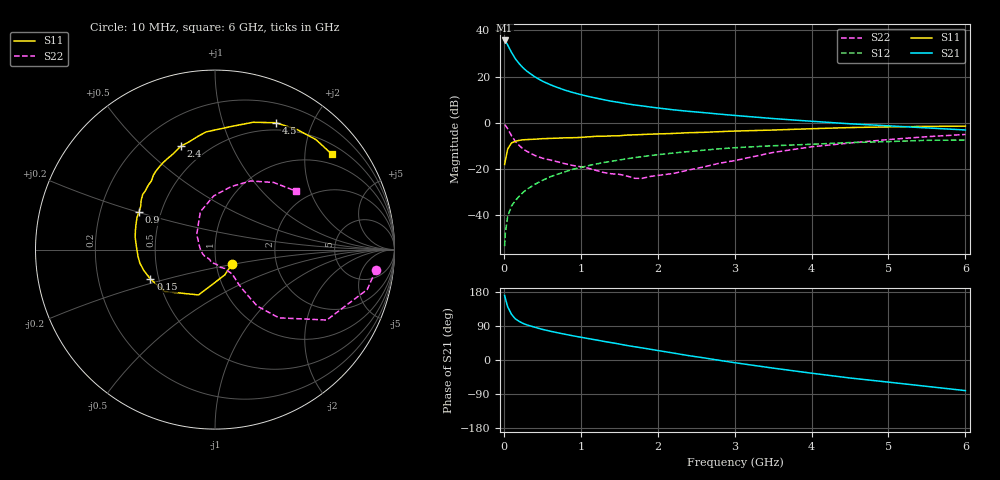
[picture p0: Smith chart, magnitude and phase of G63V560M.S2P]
! SIEMENS Small Signal Semiconductors
! BFG193
! Si NPN RF Bipolar Junction Transistor in SOT223
! VCE = 3.5 V  IC = 60 mA
! Common Emitter S-Parameters:  August  1996
# GHz  S  MA  R  50
!  f  S11  S21  S12  S22
! GHz  MAG  ANG  MAG  ANG  MAG  ANG  MAG  ANG
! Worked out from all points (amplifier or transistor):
!   36 points, 10 MHz to 6 GHz, reference 50 ohm
!   highest |S21| = 35.7 dB at 10 MHz (marker M1)
!   |S21| within 3 dB of that: start of sweep to 65.8 MHz
!   unconditionally stable (mu >= 1): 374.2 MHz to 2.36 GHz
!   at 250 MHz: K = 0.94, MSG = 27.0 dB, |S12| = -30.2 dB
!   at 1.4 GHz: K = 1.05, MAG = 11.7 dB, |S12| = -16.7 dB
!   at 6 GHz: K = 0.90, MSG = 2.2 dB, |S12| = -7.5 dB
!   S11 on the Smith chart (normalised r, x): 10 MHz: 1.20, -0.19; 150 MHz: 0.45, -0.17; 900 MHz: 0.37, +0.20; 2.4 GHz: 0.36, +0.66; 4.5 GHz: 0.41, +1.51; 6 GHz: 0.72, +2.62
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0.01  0.1243 -38.9  60.7 170.5  0.0021 85.1  0.904 -7.2
0.02  0.1516 -69.2  58.49 162.1  0.0041 80.7  0.8767 -14.7
0.05  0.2685 -109.9  48.3 140.4  0.0093 73.3  0.7363 -32.2
0.1  0.3646 -140.2  33.37 120.5  0.0156 69.3  0.5208 -46.9
0.15  0.3951 -155.5  24.27 108.4  0.0205 67.5  0.3926 -53.2
0.2  0.4136 -163.7  19.03 101.8  0.0254 70.7  0.3212 -54.3
0.25  0.4253 -169.8  15.48 96.5  0.0309 69.8  0.2679 -55.2
0.3  0.4305 -174.8  13.08 92.6  0.0359 70.5  0.2393 -55.7
0.4  0.4379 178.0  9.943 86.6  0.0458 70.7  0.1954 -55.2
0.5  0.4499 171.3  7.975 80.9  0.0559 69.6  0.1703 -54.9
0.6  0.4562 166.5  6.707 76.2  0.0668 68.4  0.1555 -56.1
0.7  0.4623 162.1  5.77 71.8  0.0765 66.8  0.1419 -58.6
0.9  0.4728 153.7  4.503 63.8  0.0978 63.1  0.1179 -62.6
1.1  0.4935 146.6  3.703 56.5  0.1173 59.6  0.1026 -73.4
1.3  0.5082 139.6  3.148 49.2  0.1369 55.3  0.0829 -83.4
1.6  0.5382 129.6  2.563 38.3  0.1651 48.5  0.0697 -109.8
2.2  0.5839 113.1  1.906 18.5  0.2195 34.7  0.0791 -175.3
2.4  0.6067 108.3  1.765 11.6  0.2363 30.4  0.0939 162.2
3.5  0.6926 82.3  1.229 -21.4  0.3161 3.1  0.2263 111.1
4.5  0.7838 64.4  0.946 -47.5  0.3706 -16.9  0.3629 75.5
5.5  0.8316 47.5  0.771 -69.6  0.4149 -40.4  0.4969 48.8
6  0.8403 39.3  0.695 -80.8  0.4198 -53.8  0.5559 35.9
